FUNCTION_BLOCK SDOwrite
VAR_INPUT
   ADSNetID:STRING(23);   (* The AMSNetID addresses the EL6751. Can be empty if only one local single channel card is present*)
   PortNr:WORD;           (* The Port No. addresses the CANopen Node (see System Manager) *)
   CO_Index:DWORD;        (* This is the Index of the CANopen Object Dictionary Entry*)
   CO_SubIndex:DWORD;     (*This is the Sub-Index of the CANopen Object Dictionary Entry*)
   DataLength:DWORD;      (* This is the Length of the CANopen Object Dictionary Entry*)
   StartWriting:BOOL;     (*only reset to FALSE after WriteDataFinished=TRUE*)
   WriteData:ARRAY[0..255] OF BYTE; (*This array contains the data to be written to the CANopen Object Dictionary*)
END_VAR
VAR_OUTPUT
   WriteDataFinished:BOOL;
   Error:DWORD;
END_VAR
VAR
   state:BYTE := 0;
   ADSWRITE:ADSWRITE;
END_VAR

CASE
state OF
   0:
        IF StartWriting THEN
           WriteDataFinished := FALSE;
           Error := 0;
           ADSWrite(
               NETID:= ADSNetID,
               PORT:= PortNr,
               IDXGRP:= CO_Index,
               IDXOFFS:= CO_SubIndex,
               LEN:= DataLength,
               SRCADDR:= ADR(WriteData),
               WRITE:= TRUE,
               TMOUT := T#1s
               );
           IF ADSWrite.err THEN
               state := 2;
               WriteDataFinished := TRUE;
               Error := ADSWrite.ErrId;
           ELSE
               state := 1;
           END_IF
        ELSE
           ADSWrite(
               NETID:= '',
               PORT:= PortNr,
               IDXGRP:= CO_Index,
               IDXOFFS:= CO_SubIndex,
               LEN:= DataLength,
               SRCADDR:= ADR(WriteData),
               WRITE:= FALSE,
               TMOUT := T#1s
               );
        END_IF
   1:
        ADSWrite(WRITE:= FALSE);
        IF ADSWrite.err THEN
           state := 2;
           WriteDataFinished := TRUE;
           Error := ADSWrite.ErrId;
        ELSE
           IF NOT ADSWrite.busy THEN
               state := 2;
               WriteDataFinished := TRUE;
           END_IF
        END_IF
   2:
        ADSWrite(WRITE:= FALSE);
        state := 0;
END_CASE

END_FUNCTION_BLOCK
